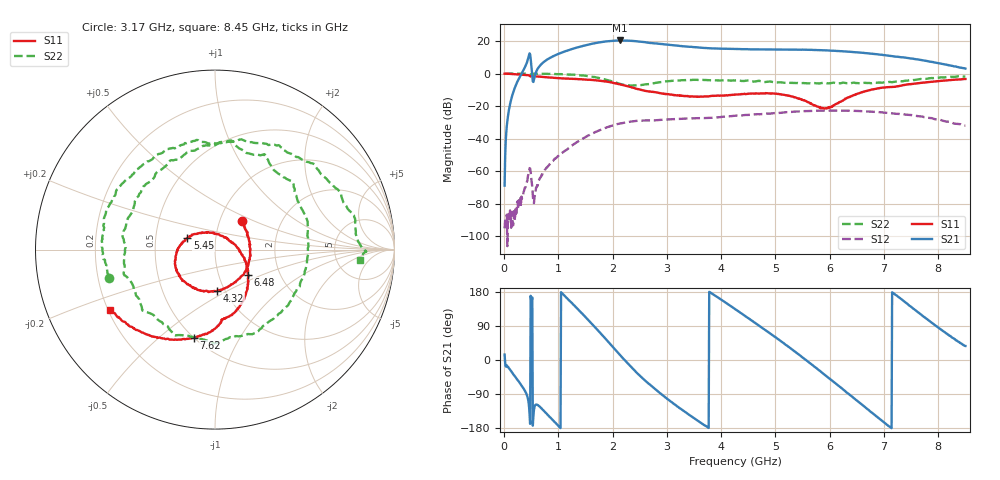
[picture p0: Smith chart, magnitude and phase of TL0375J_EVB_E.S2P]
!Agilent Technologies,E5071C,MY46523237,B.13.01
!Date: Thu Dec 21 15:42:53 2023
!Data & Calibration Information:
!Freq	S11:SOLT2(ON)	S21:SOLT2(ON)	S12:SOLT2(ON)	S22:SOLT2(ON)
!PortZ  Port1:50+j0  Port2:50+j0
!Above PortZ is port z conversion or system Z0 setting when saving the data.
!When reading, reference impedance value at option line is always used.
# Hz S dB R 50
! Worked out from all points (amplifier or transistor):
!   850 points, 10 MHz to 8.5 GHz, reference 50 ohm
!   highest |S21| = 20.4 dB at 2.14 GHz (marker M1)
!   |S21| within 3 dB of that: 1.499 GHz to 3.123 GHz (1.624 GHz wide, 70.3 % of centre)
!   unconditionally stable (mu >= 1): 15.11 MHz to 57.09 MHz; 182.2 MHz to 335.8 MHz; 366.5 MHz to end of sweep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
!   at 1.42 GHz: K = 1.46, MAG = 24.7 dB, |S12| = -40.6 dB
!   at 4.26 GHz: K = 1.18, MAG = 17.9 dB, |S12| = -25.8 dB
!   at 8.5 GHz: K = 2.33, MAG = 11.1 dB, |S12| = -32.0 dB
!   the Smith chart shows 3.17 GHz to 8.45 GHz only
!   S11 on the Smith chart (normalised r, x): 3.17 GHz: 1.27, +0.42; 4.32 GHz: 0.92, -0.45; 5.45 GHz: 0.73, +0.10; 6.48 GHz: 1.38, -0.41; 7.62 GHz: 0.50, -0.66; 8.45 GHz: 0.21, -0.25
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1e7  -0.07 -1.7  -68.90 14.4  -95.16 75.8  0.05 -1.2
4.3e8  -0.94 -59.6  7.74 -96.5  -65.66 -172.3  -0.15 -57.7
5.2e8  -1.66 -69.0  -2.22 165.1  -69.75 69.3  -0.18 -66.3
8.5e8  -2.42 -105.7  9.72 -151.4  -55.19 166.2  -0.17 -110.7
1.16e9  -3.12 -137.5  13.98 163.2  -46.60 133.7  -0.57 -151.8
1.43e9  -3.52 -165.3  16.81 123.6  -40.38 102.0  -1.13 169.1
1.79e9  -4.48 156.2  19.33 68.4  -34.42 54.1  -2.98 108.1
2.14e9  -6.70 119.9  20.38 12.4  -30.68 3.3  -6.33 27.4
2.48e9  -9.66 93.6  19.73 -38.3  -29.04 -43.0  -7.10 -62.3
2.84e9  -11.85 71.5  18.40 -83.7  -28.52 -82.6  -5.42 -125.7
3.17e9  -13.25 46.7  17.25 -119.8  -27.93 -116.0  -4.31 -165.1
3.64e9  -14.15 -2.0  15.90 -167.3  -27.38 -159.6  -3.92 150.2
4.26e9  -12.93 -81.4  15.14 133.7  -25.85 147.9  -4.22 102.2
4.32e9  -12.74 -87.3  15.06 127.9  -25.82 142.8  -4.23 98.6
4.86e9  -12.10 -140.4  14.79 74.1  -24.63 93.8  -4.97 43.5
5.45e9  -15.56 157.5  14.72 12.4  -23.27 36.8  -5.93 -28.9
5.67e9  -18.73 125.6  14.60 -12.1  -22.94 14.3  -5.86 -60.8
6.48e9  -12.69 -37.5  13.10 -104.9  -22.94 -70.8  -5.79 -168.7
7.09e9  -8.25 -81.1  10.98 -174.7  -24.20 -135.1  -5.16 117.5
7.62e9  -5.96 -103.4  8.74 127.1  -26.14 170.6  -3.69 62.9
8.45e9  -3.40 -150.4  3.46 40.5  -31.88 98.2  -1.82 -4.1
8.5e9  -3.31 -153.6  3.10 37.0  -32.01 91.8  -1.79 -9.4
